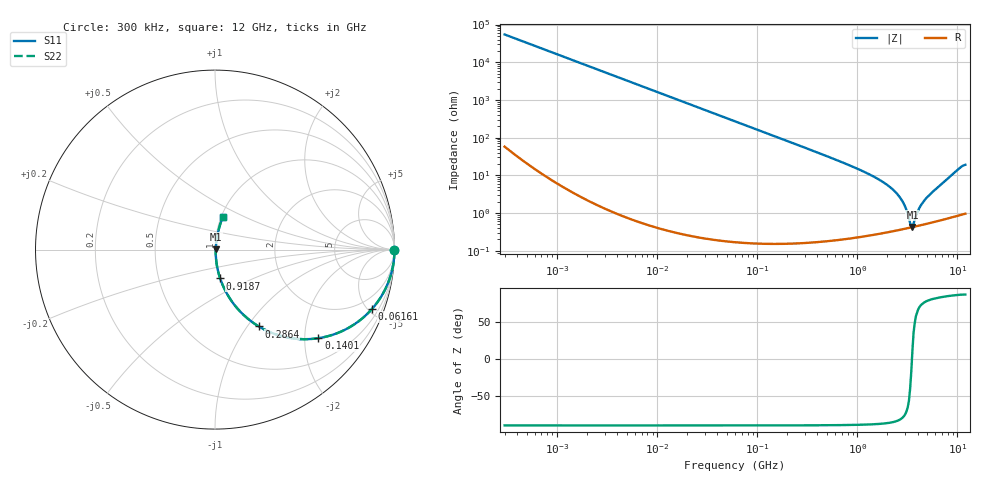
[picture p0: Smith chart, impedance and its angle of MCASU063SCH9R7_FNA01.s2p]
! MCASU063SCH9R7_FNA01  S-PARAMETER MODEL  ( General Type )
! Model Generated by TAIYO YUDEN Corporation (http://www.ty-top.com)
! Version 2.0
! TAIYO YUDEN Control No. 141022
! Copyright(c) 2013 TAIYO YUDEN CO.,LTD. All Rights Reserved.
! Product Description (link to TY-COMPAS)
! https://ds.yuden.co.jp/TYCOMPAS/or/detail?pn=MCASU063SCH9R7DFNA01&u=M
! Products Name : Multilayer Ceramic Capacitors
! Characteristics :
!  Capacitance : 9.7 pF , Rated Voltage : 50V , TCC : CH / C0H
!  Case Size : 0.6 x 0.3 / 0.024 x 0.012 [mm/inch] , Thickness : 0.3 / 0.012 [mm/inch]
!  (Conditions: Temperature = 25 degC , DC Bias Current/Voltage = 0A / 0V)
! External Node Assignments :
!  1  o---| |---o  2
! GND o---------o GND
! Frequency Range : 0.3MHz  -  12000MHz  [ 401 STEP ]
# MHz S RI R 50
! Freq[MHz].  S11 Real  S11 Imag  S21 Real  S21 Imag  S12 Real  S12 Imag  S22 Real  S22 Imag
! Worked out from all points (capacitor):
!   401 points, 300 kHz to 12 GHz, reference 50 ohm
!   read as one part in series: C = 9.74 pF near 316.3 kHz
!   lowest |Z| = 431 mohm at 3.548 GHz (marker M1)
!   series resonance near 3.513 GHz, so ESL is about 210 pH
!   S11 on the Smith chart (normalised r, x): 300 kHz: open; 61.61 MHz: 1.00, -5.30; 140.1 MHz: 1.00, -2.33; 286.4 MHz: 1.00, -1.13; 918.7 MHz: 1.00, -0.33; 12 GHz: 1.02, +0.38
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0.3  1 -0.00184  5.31e-06 0.00184  5.31e-06 0.00184  1 -0.00184
1.769972  0.9999 -0.0108  0.00012 0.0108  0.00012 0.0108  0.9999 -0.0108
10.44266  0.9959 -0.0636  0.00408 0.0636  0.00408 0.0636  0.9959 -0.0636
26.39317  0.9745 -0.1574  0.0255 0.1574  0.0255 0.1574  0.9745 -0.1574
60  0.881 -0.3234  0.119 0.3234  0.119 0.3234  0.881 -0.3234
61.61074  0.8754 -0.33  0.1246 0.33  0.1246 0.33  0.8754 -0.33
140.0606  0.5757 -0.4936  0.4243 0.4936  0.4243 0.4936  0.5757 -0.4936
286.3882  0.2438 -0.428  0.7562 0.428  0.7562 0.428  0.2438 -0.428
353.9943  0.1737 -0.377  0.8263 0.377  0.8263 0.377  0.1737 -0.377
918.7169  0.0287 -0.1605  0.9713 0.1605  0.9713 0.1605  0.0287 -0.1605
1480.043  0.0107 -0.0894  0.9893 0.0894  0.9893 0.0894  0.0107 -0.0894
2088.533  0.00565 -0.0499  0.9944 0.0499  0.9944 0.0499  0.00565 -0.0499
2448.343  0.00456 -0.0338  0.9954 0.0338  0.9954 0.0338  0.00456 -0.0338
2795.104  0.00412 -0.0209  0.9959 0.0209  0.9959 0.0209  0.00412 -0.0209
3026.31  0.00403 -0.0134  0.996 0.0134  0.996 0.0134  0.00403 -0.0134
3364.605  0.0041 -0.0035  0.9959 0.0035  0.9959 0.0035  0.0041 -0.0035
3547.679  0.00422 0.000794  0.9958 -0.000794  0.9958 -0.000794  0.00422 0.000794
3642.919  0.00429 0.00302  0.9957 -0.00302  0.9957 -0.00302  0.00429 0.00302
4270.516  0.00493 0.0145  0.9951 -0.0145  0.9951 -0.0145  0.00493 0.0145
5006.236  0.00589 0.0258  0.9941 -0.0258  0.9941 -0.0258  0.00589 0.0258
10236.47  0.029 0.1412  0.971 -0.1412  0.971 -0.1412  0.029 0.1412
12000  0.0438 0.1809  0.9562 -0.1809  0.9562 -0.1809  0.0438 0.1809
